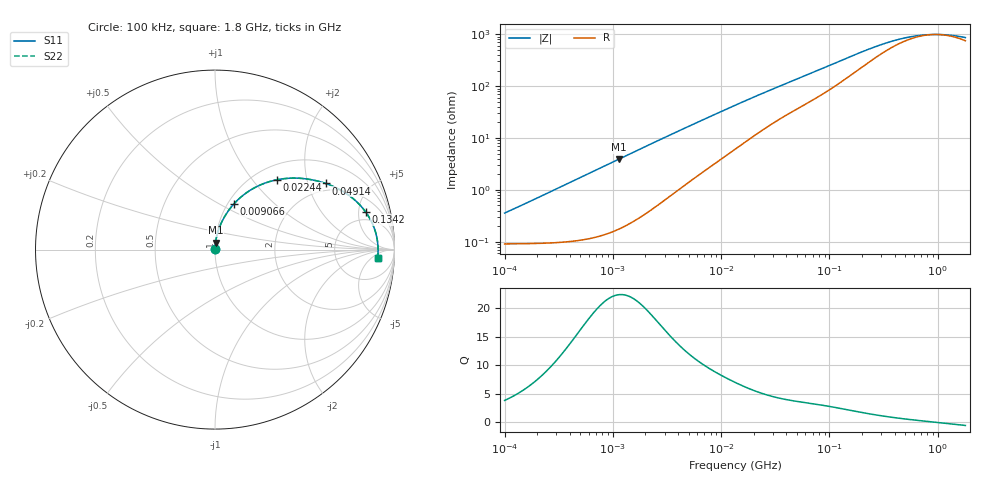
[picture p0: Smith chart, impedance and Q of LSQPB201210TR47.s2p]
! LSQPB201210TR47  S-PARAMETER MODEL  ( General Type )
! Model Generated by TAIYO YUDEN Corporation (http://www.ty-top.com)
! Version 2.0
! TAIYO YUDEN Control No. 100810NC14SB-FKC
! Copyright(c) 2008 TAIYO YUDEN CO.,LTD. All Rights Reserved.
! Product Description (link to TY-COMPAS)
! https://ds.yuden.co.jp/TYCOMPAS/or/detail?pn=LSQPB201210TR47M&u=M
! Products Name : Inductors
! Characteristics :
!  Inductance : 0.47 uH , SRF(min) : 350 MHz , DC Resistance(max) : 0.117 Ohm
!  Rated Current : Saturation :1100 mA , Temp Rise : 1050 mA (40 degC)
!  Case Size : 2.0 x 1.25 / 0.079 x 0.049 [mm/inch] , Thickness : 1.0 / 0.04 [mm/inch]
!  (Conditions: Temperature = 25 degC , DC Bias Current/Voltage = 0A / 0V)
! External Node Assignments :
!  1  o---GGG---o  2
! GND o---------o GND
! Frequency Range : 0.1MHz  -  1800MHz  [ 402 STEP ]
# MHz S RI R 50
! Freq[MHz].  S11 Real  S11 Imag  S21 Real  S21 Imag  S12 Real  S12 Imag  S22 Real  S22 Imag
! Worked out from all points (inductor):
!   401 points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, 100 kHz to 1.8 GHz, reference 50 ohm
!   read as one part in series: L = 550 nH near 105 kHz
!   highest Q = 22.3 at 1.13 MHz (marker M1), where L = 549 nH
!   self-resonance near 949.2 MHz
!   S11 on the Smith chart (normalised r, x): 100 kHz: 1.00, +0.01; 9.066 MHz: 1.07, +0.59; 22.44 MHz: 1.26, +1.34; 49.14 MHz: 1.71, +2.60; 134.2 MHz: 3.58, +5.98; 1.8 GHz: 16, -9
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0.1  0.000918 0.00345  0.9991 -0.00345  0.9991 -0.00345  0.000918 0.00345
0.155413  0.000944 0.00536  0.9991 -0.00536  0.9991 -0.00536  0.000944 0.00536
0.516129  0.00139 0.0178  0.9986 -0.0178  0.9986 -0.0178  0.00139 0.0178
1.130264  0.00325 0.0388  0.9968 -0.0388  0.9968 -0.0388  0.00325 0.0388
2.66389  0.0133 0.0893  0.9867 -0.0893  0.9867 -0.0893  0.0133 0.0893
5.289144  0.0439 0.1663  0.9561 -0.1663  0.9561 -0.1663  0.0439 0.1663
7.096489  0.0714 0.2118  0.9286 -0.2118  0.9286 -0.2118  0.0714 0.2118
9.066201  0.1052 0.2544  0.8948 -0.2544  0.8948 -0.2544  0.1052 0.2544
13.41641  0.1867 0.3246  0.8133 -0.3246  0.8133 -0.3246  0.1867 0.3246
17.56533  0.2639 0.3651  0.7361 -0.3651  0.7361 -0.3651  0.2639 0.3651
22.44079  0.3459 0.3893  0.6541 -0.3893  0.6541 -0.3893  0.3459 0.3893
32.40491  0.4765 0.3971  0.5235 -0.3971  0.5235 -0.3971  0.4765 0.3971
49.1428  0.6158 0.3688  0.3842 -0.3688  0.3842 -0.3688  0.6158 0.3688
69.24595  0.7133 0.3237  0.2867 -0.3237  0.2867 -0.3237  0.7133 0.3237
95.21179  0.7846 0.2709  0.2154 -0.2709  0.2154 -0.2709  0.7846 0.2709
134.1607  0.8385 0.2108  0.1615 -0.2108  0.1615 -0.2108  0.8385 0.2108
208.5031  0.8784 0.1415  0.1216 -0.1415  0.1216 -0.1415  0.8784 0.1415
357.3983  0.8997 0.0773  0.1003 -0.0773  0.1003 -0.0773  0.8997 0.0773
542.0029  0.9061 0.0404  0.0939 -0.0404  0.0939 -0.0404  0.9061 0.0404
802.0705  0.9084 0.0116  0.0916 -0.0116  0.0916 -0.0116  0.9084 0.0116
1186.925  0.9086 -0.0155  0.0914 0.0155  0.0914 0.0155  0.9086 -0.0155
1800  0.9065 -0.0471  0.0935 0.0471  0.0935 0.0471  0.9065 -0.0471
